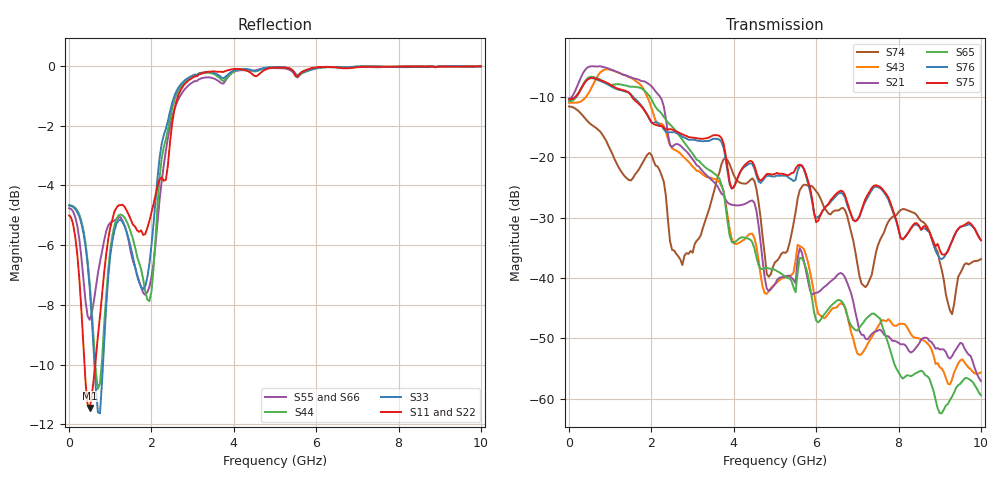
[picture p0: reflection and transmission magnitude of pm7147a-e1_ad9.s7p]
# GHz S DB R 50
! S-Parameters data
! Freq  dbS11  angS11  dbS12  angS12  dbS13  angS13  dbS14  angS14
!  dbS15  angS15  dbS16  angS16  dbS17  angS17  dbS21  angS21
!  dbS22  angS22  dbS23  angS23  dbS24  angS24  dbS25  angS25
!  dbS26  angS26  dbS27  angS27  dbS31  angS31  dbS32  angS32
!  dbS33  angS33  dbS34  angS34  dbS35  angS35  dbS36  angS36
!  dbS37  angS37  dbS41  angS41  dbS42  angS42  dbS43  angS43
!  dbS44  angS44  dbS45  angS45  dbS46  angS46  dbS47  angS47
!  dbS51  angS51  dbS52  angS52  dbS53  angS53  dbS54  angS54
!  dbS55  angS55  dbS56  angS56  dbS57  angS57  dbS61  angS61
!  dbS62  angS62  dbS63  angS63  dbS64  angS64  dbS65  angS65
!  dbS66  angS66  dbS67  angS67  dbS71  angS71  dbS72  angS72
!  dbS73  angS73  dbS74  angS74  dbS75  angS75  dbS76  angS76
!  dbS77  angS77
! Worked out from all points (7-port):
!   279 points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, 1 Hz to 10 GHz, reference 50 ohm
!   strongest paths, dB at 1 Hz, 7.943 MHz, 3.05 GHz, 6.55 GHz, 10 GHz:
!     S75: -10.4, -10.4, -16.8, -25.7, -33.7
!     S76: -10.4, -10.4, -17.1, -26.0, -33.7
!     S65: -10.7, -10.7, -19.9, -43.6, -59.4
!     S21: -10.3, -10.3, -20.8, -39.3, -57.1
!     S43: -11.0, -11.0, -21.9, -44.5, -55.7
!     S74: -11.6, -11.6, -34.4, -28.8, -36.9
!   lowest |S11| = -11.5 dB at 500 MHz (marker M1), VSWR 1.73, Z = 28.9 - j0.835 ohm
!   |S11| at or under -10 dB: 373.9 MHz to 633.5 MHz (259.6 MHz wide, 51.5 % of centre)
